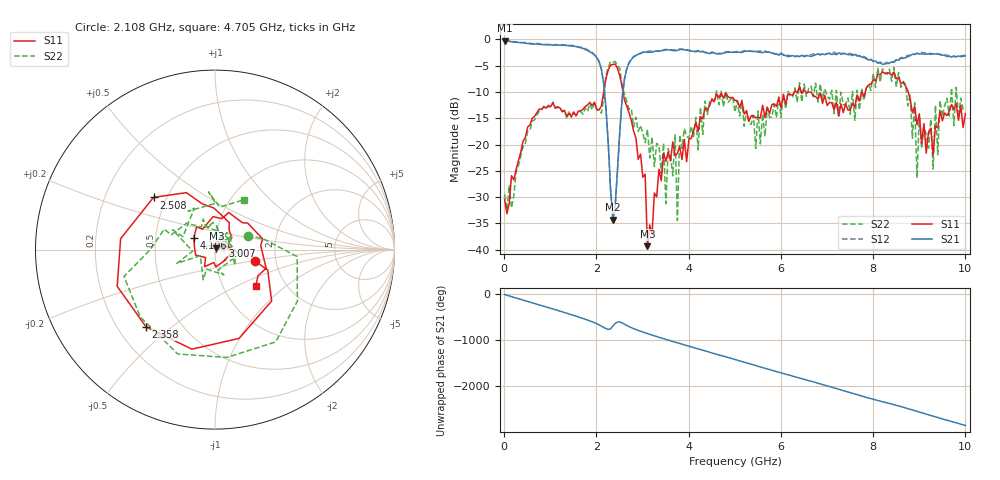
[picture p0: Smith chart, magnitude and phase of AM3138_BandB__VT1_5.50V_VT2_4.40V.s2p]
! Date/Time: Tue, Nov 13, 2018 4:40 PM
! Network Analyzer: Agilent Technologies E8364B Rev: A.07.50.67
! Sweep from 0.010 to 10.000 GHz, 201 Points, Sweep Type: LIN
! Power Supply: 5.501 V, 0.000 A
# Hz S DB R 50
!freq MagS11 AngS11 MagS21 AngS21 MagS12 AngS12 MagS22 AngS22
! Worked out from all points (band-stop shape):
!   201 points, 10 MHz to 10 GHz, reference 50 ohm
!   highest |S21| = -0.26 dB at 10 MHz (marker M1); lowest = -34.3 dB at 2.358 GHz (marker M2)
!   |S21| within 3 dB of the highest: start of sweep to 1.987 GHz; 2.825 GHz to 6.145 GHz (3.321 GHz wide, 74 % of centre)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
!   lowest |S11| = -39.3 dB at 3.107 GHz (marker M3), VSWR 1.02, Z = 50.7 + j0.799 ohm
!   |S11| at or under -10 dB: start of sweep to 2.158 GHz; 2.577 GHz to 6.292 GHz (3.715 GHz wide, 83.8 % of centre); 8.759 GHz to end of sweep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
!   |S22| runs from -34.4 to -4.2 dB; largest |S21 - S12| = 0.035
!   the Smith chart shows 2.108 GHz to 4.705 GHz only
!   S11 on the Smith chart (normalised r, x): 2.108 GHz: 1.56, -0.21; 2.358 GHz: 0.32, -0.41; 2.508 GHz: 0.42, +0.31; 3.007 GHz: 1.09, +0.05; 4.106 GHz: 0.78, +0.10; 4.705 GHz: 1.42, -0.64
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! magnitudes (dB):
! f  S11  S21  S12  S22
! 10 MHz  -30.5  -0.3  -0.2  -29.4
! 1.708 GHz  -13.3  -1.7  -1.6  -14.3
! 2.108 GHz  -12.7  -5.6  -5.6  -14.1
! 2.358 GHz  -4.8  -34.3  -34.0  -4.4
! 2.508 GHz  -6.9  -17.6  -17.5  -5.5
! 3.007 GHz  -26.2  -2.5  -2.4  -17.9
! 3.107 GHz  -39.3  -2.4  -2.3  -17.1
! 3.357 GHz  -24.7  -2.3  -2.2  -20.1
! 3.507 GHz  -23.2  -2.0  -1.9  -31.2
! 3.706 GHz  -22.1  -2.2  -2.0  -18.1
! 3.756 GHz  -21.7  -2.1  -2.0  -34.4
! 3.806 GHz  -20.4  -2.0  -1.8  -18.2
! 4.106 GHz  -17.4  -2.3  -2.3  -18.5
! 4.705 GHz  -10.3  -2.8  -2.7  -9.9
! 5.005 GHz  -11.6  -2.4  -2.4  -13.8
! 6.703 GHz  -10.7  -3.1  -2.8  -10.9
! 8.352 GHz  -6.4  -4.6  -4.6  -5.7
! 8.901 GHz  -12.7  -2.8  -2.9  -12.1
! 8.951 GHz  -16.2  -2.7  -2.7  -26.4
! 9.001 GHz  -14.2  -2.8  -2.7  -14.2
! 9.301 GHz  -22.0  -2.7  -2.7  -24.6
! 10 GHz  -14.1  -3.1  -3.1  -13.4
